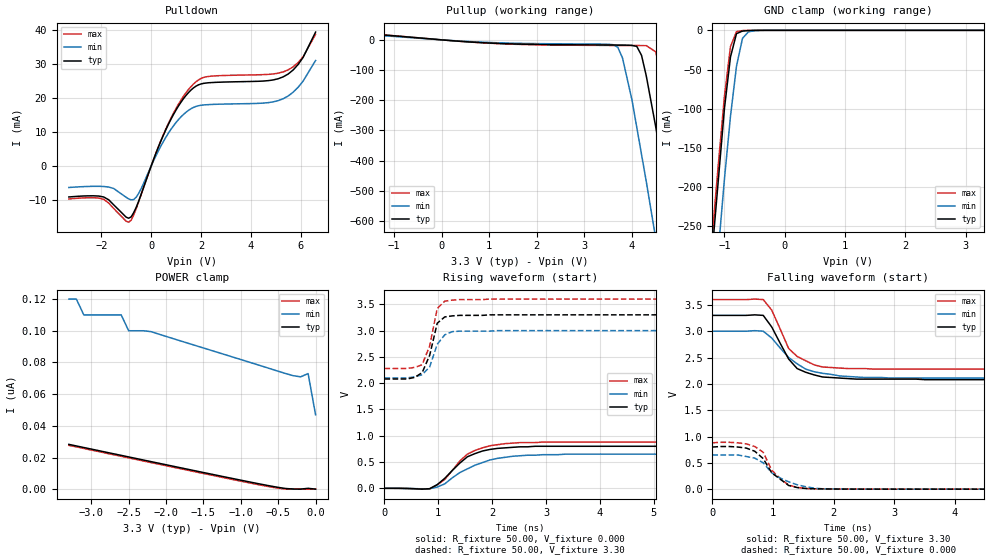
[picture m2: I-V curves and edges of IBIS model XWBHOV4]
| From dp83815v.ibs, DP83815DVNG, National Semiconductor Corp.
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|   Model XWBHOV4
[Model]   XWBHOV4
Model_type   I/O
Polarity   Non-Inverting
Enable   Active-High
Vinl =   0.80V
Vinh =   2.00V
Vmeas =   1.50V
Cref =  20.00pF
Rref = 100.00k
C_comp   5.00pF   5.00pF   5.00pF
[Temperature Range]   25.00   0.14k   0.000
[Voltage Range]   3.30V   3.00V   3.60V
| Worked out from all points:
|   slope of the pulldown table from 0 to 0.495 V, typ, clamps not added: 54 ohm
|   slope of the pullup table from 0 to 0.495 V, typ, clamps not added: 83 ohm
|   GND clamp passes 1 mA (typ) near -0.70 V on its own axis
|   rising waveform, R_fixture 50.00, V_fixture 0.000: 20-80 % time 549ps typ, 729ps min, 523ps max; typ from 0 V to 0.8 V
|   rising waveform, R_fixture 50.00, V_fixture 3.30: 20-80 % time 208ps typ, 230ps min, 188ps max; typ from 2.08 V to 3.3 V
|   falling waveform, R_fixture 50.00, V_fixture 3.30: 20-80 % time 383ps typ, 523ps min, 373ps max; typ from 3.3 V to 2.08 V
|   falling waveform, R_fixture 50.00, V_fixture 0.000: 20-80 % time 375ps typ, 476ps min, 312ps max; typ from 0.8 V to 0 V
[Pulldown]
| voltage   I(typ)   I(min)   I(max)
-3.3V     -9.06mA    -6.27mA    -9.65mA
-1.9V     -9.07mA    -5.98mA    -9.76mA
-900mV    -15.32mA   -9.63mA    -16.49mA
-700mV    -13.7mA    -9.83mA    -14.39mA
-500mV    -10.32mA   -8.02mA    -10.47mA
700mV     12.41mA    9.79mA     12.68mA
1.2V      18.87mA    14.53mA    19.49mA
1.7V      23.06mA    17.31mA    24.2mA
2.3V      24.57mA    18.14mA    26.43mA
5.3V      26.32mA    19.87mA    27.77mA
5.9V      29.96mA    23.25mA    30.53mA
6.6V      39.5mA     31.14mA    38.86mA
[Pullup]
| voltage   I(typ)   I(min)   I(max)
-3.3V     5.74mA     3.42mA     12.88mA
-2.7V     30.03mA    6.6mA      32.05mA
3.6V      -17.13mA   -15.98mA   -18.55mA
3.8V      -17.31mA   -60.1mA    -18.69mA
4.1V      -21.65mA   -290mA     -18.88mA
4.3V      -120mA     -470mA     -19.31mA
4.5V      -290mA     -660mA     -39.95mA
4.7V      -480mA     -850mA     -190mA
4.9V      -680mA     -1.05A     -370mA
5.1V      -870mA     -1.24A     -560mA
5.3V      -1.07A     -1.44A     -760mA
6.6V      -2.36A     -2.73A     -2.05A
[GND_clamp]
| voltage   I(typ)   I(min)   I(max)
-3.3V     -2.34A     -2.41A     -2.33A
-1.2V     -280mA     -370mA     -260mA
-1.1V     -190mA     -280mA     -170mA
-1V       -100mA     -190mA     -84.34mA
-900mV    -34.08mA   -110mA     -20.85mA
-800mV    -4.23mA    -45.82mA   -1.68mA
-700mV    -960uA     -10.12mA   -320uA
-600mV    -330uA     -1.84mA    -56.62uA
-500mV    -61.49uA   -550uA     -4.93uA
3.3V      60.66pA    71.66nA    35.7pA
[POWER_clamp]
| voltage   I(typ)   I(min)   I(max)
-3.3V     28.3nA     120nA      27.7nA
-3.2V     27.31nA    120nA      26.71nA
-3.1V     26.32nA    110nA      25.72nA
-2.6V     21.37nA    110nA      20.76nA
-2.5V     20.38nA    100nA      19.77nA
-2.2V     17.41nA    99.43nA    16.81nA
-600mV    2nA        75.94nA    1.42nA
-400mV    460pA      73nA       140pA
-300mV    110pA      71.66nA    300pA
-200mV    76.73pA    70.92nA    74.52pA
-100mV    570pA      72.98nA    41.38pA
0V        60.66pA    46.97nA    39.08pA
[Ramp]
| variable   typ   min   max
dV/dt_r   1.70/0.43n   1.50/0.57n   1.86/0.42n
dV/dt_f   1.79/0.29n   1.59/0.42n   1.96/0.28n
R_load = 0.50k
[Rising Waveform]
R_fixture = 50.00
V_fixture = 0.000
V_fixture_min = 0.000
V_fixture_max = 0.000
| time   V(typ)   V(min)   V(max)
0s        160uV      130uV      170uV
840ps     -7.03mV    -7.74mV    -9.29mV
980ps     70.85mV    25.09mV    64.8mV
1.12ns    190mV      84.52mV    170mV
1.4ns     480mV      300mV      520mV
1.54ns    600mV      370mV      650mV
1.82ns    710mV      490mV      770mV
2.24ns    770mV      590mV      850mV
3.36ns    800mV      650mV      880mV
7ns       800mV      650mV      880mV
[Rising Waveform]
R_fixture = 50.00
V_fixture = 3.30
V_fixture_min = 3.00
V_fixture_max = 3.60
| time   V(typ)   V(min)   V(max)
0s        2.08V      2.1V       2.28V
420ps     2.08V      2.1V       2.28V
560ps     2.11V      2.12V      2.3V
700ps     2.2V       2.16V      2.35V
840ps     2.53V      2.31V      2.71V
980ps     3.14V      2.74V      3.42V
1.12ns    3.26V      2.92V      3.56V
1.26ns    3.28V      2.98V      3.58V
2.1ns     3.3V       3V         3.6V
7ns       3.3V       3V         3.6V
[Falling Waveform]
R_fixture = 50.00
V_fixture = 3.30
V_fixture_min = 3.00
V_fixture_max = 3.60
| time   V(typ)   V(min)   V(max)
0s        3.3V       3V         3.6V
840ps     3.3V       3V         3.6V
980ps     3.08V      2.87V      3.4V
1.26ns    2.47V      2.5V       2.67V
1.4ns     2.29V      2.38V      2.52V
1.54ns    2.22V      2.28V      2.44V
1.82ns    2.13V      2.2V       2.32V
2.1ns     2.11V      2.15V      2.3V
2.94ns    2.09V      2.11V      2.28V
7ns       2.08V      2.1V       2.28V
[Falling Waveform]
R_fixture = 50.00
V_fixture = 0.000
V_fixture_min = 0.000
V_fixture_max = 0.000
| time   V(typ)   V(min)   V(max)
0s        800mV      650mV      880mV
420ps     800mV      650mV      880mV
700ps     720mV      590mV      810mV
840ps     580mV      500mV      700mV
980ps     310mV      310mV      360mV
1.12ns    190mV      210mV      200mV
1.26ns    69.82mV    140mV      77.01mV
1.54ns    13.44mV    47.16mV    11.19mV
2.1ns     1.92mV     3.02mV     1.78mV
7ns       4.79uV     8.66uV     2.88uV
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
